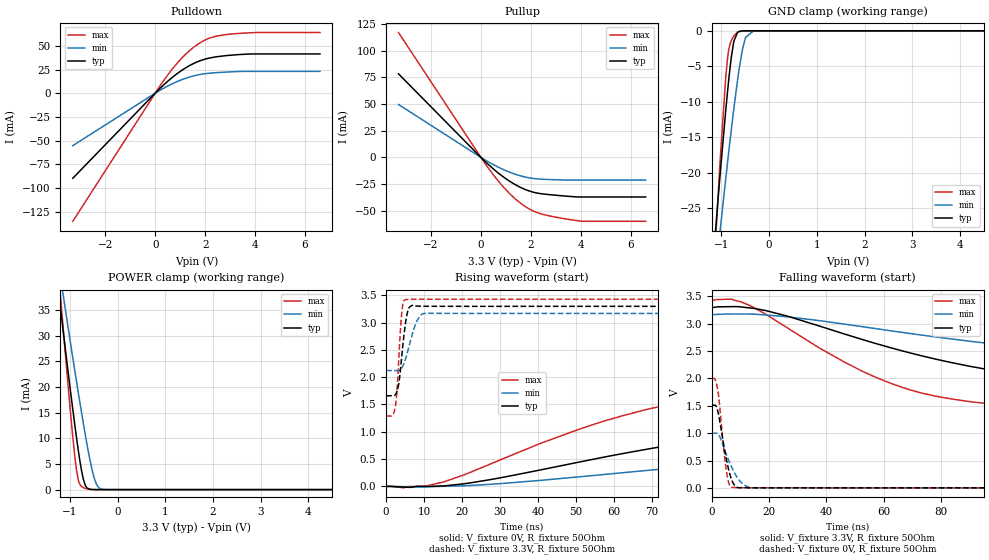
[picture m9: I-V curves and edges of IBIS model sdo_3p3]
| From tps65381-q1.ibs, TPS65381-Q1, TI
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|   sdo_3p3 Model
[Model]   sdo_3p3
Model_type   I/O
Polarity   Non-Inverting
Enable   Active-High
Vinl = 0.99
Vinh = 2.31
Vmeas = 1.65
Vref = 0
Cref = 100pF
Rref = 100
|   typ   min   max
|   (nom PVT)   (fast PVT)   (slow PVT)
C_comp   1.636e-12   1.597e-12   1.694e-12
[Model spec]
|subparameter
Vinl   0.99   0.951   1.029
Vinh   2.31   2.219   2.401
| Where nom  PVT is Nominal Process, 3.3V, 27C
|   Fast PVT is Strong Process,  3.43V, -40C
|   Slow PVT is Weak Process,   3.17V, 150C
[Voltage Range]   3.3   3.17   3.43
|Junction Temperature
[Temperature Range]   27   150   -40
[Pullup Reference]   3.3   3.17   3.43
[Pulldown Reference]   0   0   0
[Power Clamp Reference]   3.3   3.17   3.43
[GND Clamp Reference]   0   0   0
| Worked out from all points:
|   slope of the pulldown table from 0 to 0.495 V, typ, clamps not added: 39.8 ohm
|   slope of the pullup table from 0 to 0.495 V, typ, clamps not added: 46.2 ohm
|   GND clamp passes 1 mA (typ) near -0.71 V on its own axis
|   POWER clamp passes 1 mA (typ) near -0.69 V on its own axis
|   falling waveform, V_fixture 3.3V, R_fixture 50Ohm: 20-80 % time 84.2ns typ, 123ns min, 50.7ns max; typ from 3.3 V to 1.66 V
|   rising waveform, V_fixture 0V, R_fixture 50Ohm: 20-80 % time 90.2ns typ, 131ns min, 55.4ns max; typ from 0 V to 1.51 V
|   rising waveform, V_fixture 3.3V, R_fixture 50Ohm: 20-80 % time 1.53ns typ, 2.62ns min, 1.09ns max; typ from 1.66 V to 3.3 V
|   falling waveform, V_fixture 0V, R_fixture 50Ohm: 20-80 % time 3.22ns typ, 4.99ns min, 2.31ns max; typ from 1.51 V to 0 V
[Pulldown]
|   Voltage   I(typ)   I(min)   I(max)
-3.3V     -89.83mA   -55.4mA    -135.3mA
253.6mV   6.633mA    4.012mA    10.12mA
637.1mV   15.64mA    9.371mA    23.92mA
932.6mV   21.68mA    12.88mA    33.24mA
1.254V    27.28mA    16.05mA    41.99mA
1.605V    32.17mA    18.7mA     49.78mA
1.946V    35.59mA    20.4mA     55.46mA
2.174V    37.14mA    21.09mA    58.14mA
2.871V    39.77mA    22.34mA    62.02mA
4.001V    41.46mA    23.03mA    64.03mA
6.6V      41.46mA    23.03mA    64.03mA
[GND Clamp]
|   Voltage   I(typ)   I(min)   I(max)
-3.3V     -239.8mA   -194.8mA   -331.5mA
-1.18V    -32.91mA   -38.03mA   -36.41mA
-1.046V   -21.78mA   -29.36mA   -20.52mA
-1.023V   -19.92mA   -27.9mA    -17.92mA
-909.3mV  -11.24mA   -20.84mA   -6.541mA
-868.1mV  -8.347mA   -18.36mA   -3.685mA
-825mV    -5.568mA   -15.82mA   -2mA
-739.2mV  -1.472mA   -10.97mA   -711.2uA
-643.5mV  -146.2uA   -6.09mA    -134uA
-494.5mV  -2.671uA   -948.5uA   -1.937uA
-330mV    -16.59nA   -26.17uA   0A
6.6V      0A         0A         0A
[Pullup]
|   Voltage   I(typ)   I(min)   I(max)
-3.3V     78.34mA    49.61mA    117.1mA
227.7mV   -5.129mA   -3.232mA   -7.763mA
678.4mV   -14.3mA    -8.947mA   -21.67mA
922.3mV   -18.67mA   -11.63mA   -28.33mA
1.254V    -23.87mA   -14.78mA   -36.3mA
1.585V    -28.13mA   -17.28mA   -42.92mA
1.965V    -31.72mA   -19.29mA   -48.71mA
2.332V    -33.77mA   -20.32mA   -52.36mA
2.867V    -35.22mA   -20.86mA   -55.46mA
3.633V    -36.71mA   -21.27mA   -58.54mA
4.143V    -37.13mA   -21.27mA   -59.92mA
6.6V      -37.13mA   -21.27mA   -59.92mA
[POWER Clamp]
|   Voltage   I(typ)   I(min)   I(max)
-3.3V     205.9mA    175mA      284.1mA
-1.227V   37.42mA    43.07mA    40.83mA
-1.17V    32.98mA    39.57mA    34.45mA
-1.144V   30.99mA    38mA       31.61mA
-947mV    16.05mA    26.02mA    10.8mA
-861.3mV  9.992mA    20.95mA    3.704mA
-792.7mV  5.612mA    16.98mA    1.023mA
-679.8mV  845.4uA    10.72mA    238.4uA
-485mV    6.263uA    2.03mA     2.016uA
-393.1mV  486.7nA    340.9uA    70.37nA
-320.2mV  52.3nA     53.53uA    0A
6.6V      0A         0A         0A
[Ramp]
R_load = 50
|   typ   min   max
dV/dt_r   0.90681/9.00516e-08   0.598989/1.30919e-07   1.1999/5.51625e-08
dV/dt_f   0.984088/8.41734e-08   0.628491/1.22823e-07   1.28501/5.05554e-08
[Falling Waveform]
V_fixture = 3.3V
V_fixture_min = 3.17V
V_fixture_max = 3.43V
R_fixture = 50Ohm
|   Time   V(typ)   V(min)   V(max)
0s        3.3V       3.17V      3.43V
6.975ns   3.314V     3.179V     3.451V
12.83ns   3.293V     3.179V     3.345V
46.65ns   2.808V     2.992V     2.29V
68.4ns    2.479V     2.829V     1.806V
90.8ns    2.217V     2.677V     1.572V
121.4ns   1.985V     2.513V     1.442V
174.9ns   1.805V     2.329V     1.35V
285.7ns   1.697V     2.18V      1.299V
750ns     1.66V      2.123V     1.288V
[Rising Waveform]
V_fixture = 0V
V_fixture_min = 0V
V_fixture_max = 0V
R_fixture = 50Ohm
|   Time   V(typ)   V(min)   V(max)
0s        681.8pV    203.5nV    523pV
4.725ns   -13.5mV    -5.054mV   -26.95mV
14.95ns   8.256mV    2.055mV    78.86mV
51.07ns   449mV      176.7mV    1.053V
74.23ns   747mV      327.9mV    1.496V
95.57ns   964.4mV    455.4mV    1.719V
128.7ns   1.198V     616.2mV    1.857V
184.1ns   1.383V     795.3mV    1.945V
298.4ns   1.482V     945mV      1.991V
750ns     1.511V     998.3mV    2V
[Rising Waveform]
V_fixture = 3.3V
V_fixture_min = 3.17V
V_fixture_max = 3.43V
R_fixture = 50Ohm
|   Time   V(typ)   V(min)   V(max)
0s        1.66V      2.122V     1.288V
2.3ns     1.671V     2.122V     1.419V
2.8ns     1.73V      2.121V     1.709V
3.275ns   1.865V     2.124V     2.261V
4.3ns     2.517V     2.192V     3.294V
5.125ns   3.004V     2.341V     3.42V
5.975ns   3.265V     2.554V     3.426V
8.125ns   3.303V     3.032V     3.428V
10.9ns    3.299V     3.176V     3.428V
750ns     3.3V       3.17V      3.43V
[Falling Waveform]
V_fixture = 0V
V_fixture_min = 0V
V_fixture_max = 0V
R_fixture = 50Ohm
|   Time   V(typ)   V(min)   V(max)
0s        1.511V     998.8mV    2V
1.05ns    1.513V     998.8mV    1.991V
1.925ns   1.43V      997.5mV    1.827V
2.5ns     1.299V     962.7mV    1.617V
5.15ns    503.3mV    598.1mV    285.3mV
6.15ns    275.7mV    467.7mV    53.23mV
7.35ns    94.42mV    329.2mV    6.734mV
10.65ns   3.387mV    78.6mV     1.295mV
14.65ns   799.3uV    375uV      1.607mV
750ns     31.55nV    394.6nV    3.296nV
